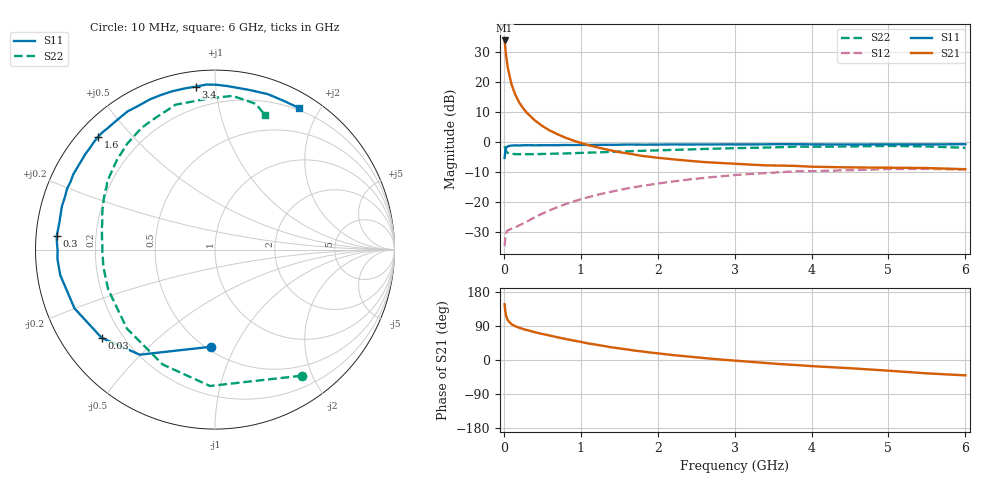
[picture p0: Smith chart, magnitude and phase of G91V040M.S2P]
! SIEMENS Small Signal Semiconductors
! BFG235
! Si NPN RF Bipolar Junction Transistor in SOT223
! VCE = 1 V  IC = 40 mA
! Common Emitter S-Parameters:  July  1994
# GHz  S  MA  R  50
!  f  S11  S21  S12  S22
! GHz  MAG  ANG  MAG  ANG  MAG  ANG  MAG  ANG
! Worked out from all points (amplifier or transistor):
!   40 points, 10 MHz to 6 GHz, reference 50 ohm
!   highest |S21| = 33.8 dB at 10 MHz (marker M1)
!   |S21| within 3 dB of that: start of sweep to 21.21 MHz
!   unconditionally stable (mu >= 1): 482 MHz to 1.574 GHz; 1.788 GHz to 1.824 GHz
!   at 200 MHz: K = 0.65, MSG = 20.4 dB, |S12| = -27.7 dB
!   at 1.5 GHz: K = 1.02, MAG = 5.5 dB, |S12| = -16.0 dB
!   at 6 GHz: K = 0.97, MSG = 0.1 dB, |S12| = -9.2 dB
!   S11 on the Smith chart (normalised r, x): 10 MHz: 0.53, -0.81; 30 MHz: 0.12, -0.34; 300 MHz: 0.06, +0.04; 1.6 GHz: 0.06, +0.40; 3.4 GHz: 0.08, +0.88; 6 GHz: 0.17, +1.74
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0.01  0.5417 -92.4  48.9 147.2  0.0185 58.4  0.8525 -55.5
0.02  0.7202 -125.6  35.82 127.5  0.0271 41.3  0.7603 -92.1
0.03  0.8002 -142.1  27.02 116.2  0.0308 32.7  0.7035 -114.4
0.05  0.8486 -157.3  17.48 105.2  0.0338 24.9  0.6592 -138.1
0.1  0.8738 -170.6  9.07 94.5  0.0361 24.4  0.6352 -159.6
0.15  0.8794 -176.5  6.076 89.0  0.038 28.2  0.6285 -168.1
0.2  0.8771 -179.6  4.54 85.2  0.0412 32.0  0.6282 -172.8
0.25  0.8815 177.4  3.658 81.8  0.0441 35.8  0.6267 -176.0
0.3  0.8853 175.1  3.056 79.0  0.0474 39.4  0.6281 -178.7
0.4  0.8801 170.8  2.306 73.6  0.0558 44.3  0.628 177.6
0.5  0.8823 166.9  1.847 68.7  0.0644 47.5  0.6325 174.5
0.6  0.8866 164.2  1.547 64.5  0.0733 49.4  0.6364 171.7
0.8  0.8913 157.7  1.182 55.6  0.0925 50.9  0.6451 166.8
1.1  0.8932 148.6  0.885 43.6  0.1209 49.6  0.6656 160.3
1.6  0.9057 136.1  0.65 27.9  0.1685 43.2  0.6981 149.8
2.2  0.9111 122.3  0.515 12.9  0.2204 33.3  0.74 137.6
3.2  0.9136 101.0  0.421 -4.7  0.2933 14.2  0.7982 117.5
3.4  0.9145 96.8  0.409 -7.8  0.3034 10.2  0.808 113.2
4.5  0.9098 77.8  0.378 -21.7  0.3398 -10.1  0.843 92.3
5  0.9148 71.3  0.374 -28.2  0.3545 -18.4  0.8619 83.5
5.5  0.9129 65.1  0.369 -35.3  0.3572 -27.8  0.8436 74.4
6  0.9171 59.5  0.353 -40.5  0.3465 -34.3  0.8007 69.7
